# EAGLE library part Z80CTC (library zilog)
Z80 FAMILY DEVICE
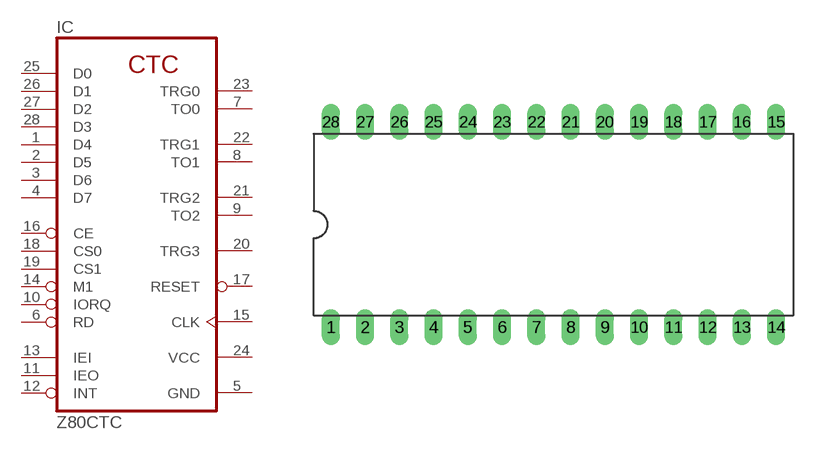
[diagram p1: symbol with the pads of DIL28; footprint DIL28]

Designator prefix IC

## Z80CTC  [DIL28]
1  D4
2  D5
3  D6
4  D7
5  GND  pwr
6  RD  in
7  TO0  out
8  TO1  out
9  TO2  out
10  IORQ  in
11  IEO  out
12  INT  out
13  IEI  in
14  M1  in
15  CLK  in
16  CE  in
17  RESET  in
18  CS0  in
19  CS1  in
20  TRG3  in
21  TRG2  in
22  TRG1  in
23  TRG0  in
24  VCC  pwr
25  D0
26  D1
27  D2
28  D3

## Footprint DIL28 (pad centres in mm)
Dual In Line Package
drill 0.813 long: 1 -16.51,-7.62; 2 -13.97,-7.62; 3 -11.43,-7.62; 4 -8.89,-7.62; 5 -6.35,-7.62; 6 -3.81,-7.62; 7 -1.27,-7.62; 8 1.27,-7.62; 9 3.81,-7.62; 10 6.35,-7.62; 11 8.89,-7.62; 12 11.43,-7.62; 13 13.97,-7.62; 14 16.51,-7.62; 15 16.51,7.62; 16 13.97,7.62; 17 11.43,7.62; 18 8.89,7.62; 19 6.35,7.62; 20 3.81,7.62; 21 1.27,7.62; 22 -1.27,7.62; 23 -3.81,7.62; 24 -6.35,7.62; 25 -8.89,7.62; 26 -11.43,7.62; 27 -13.97,7.62; 28 -16.51,7.62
